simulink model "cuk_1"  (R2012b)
settings: Solver=ode45  StartTime=0.0  StopTime=10.0  RelTol=1e-3
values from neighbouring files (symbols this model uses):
  C1 = 200e-6    (= 0.0002)    [Cuk1.m]    (also in sepic1.m = 0.0001; sepic2.m = 0.0001; feder_masse_1.m = [1 0 0 0]; feder_masse_13.m = [1 0 0 0])
  C2 = C1    (= 0.0002)    [Cuk1.m]    (also in sepic1.m = 0.0001; sepic2.m = 0.0001; feder_masse_1.m = [0 0 1 0]; feder_masse_13.m = [0 0 1 0])
  f0 = 0.2e5    (= 20000)    [boost_up1.m]    (also in buck_boost1.m; buck_boost2.m; buck_down1.m; buck_down2.m)
  L1 = 0.0001    [Cuk1.m]    (also in sepic1.m = 5e-05; sepic2.m = 5e-05)
  L2 = L1    (= 0.0001)    [Cuk1.m]    (also in sepic1.m = 5e-05; sepic2.m = 5e-05)
  R = 5    [boost_up1.m]    (also in buck_boost1.m; buck_boost2.m; buck_down1.m = 2*Rmax,; buck_down2.m = 0.1*Rmax,)
  T = 1/f0    (= 5e-05)    [boost_up1.m]    (also in buck_boost1.m; buck_boost2.m; buck_down1.m; buck_down2.m)
  T1 = T-T2    (= 2.5e-05)    [buck_boost1.m]    (also in buck_boost2.m = 1e-05; sepic1.m = T-T2; sepic2.m = T-T2; unwucht_4.m = 500)
  Ui = 5    [boost_up1.m]    (also in buck_boost1.m; buck_boost2.m; buck_down1.m; buck_down2.m)

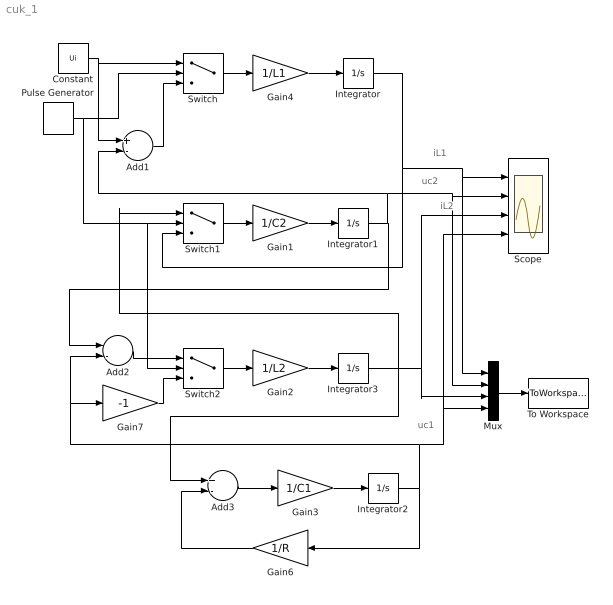
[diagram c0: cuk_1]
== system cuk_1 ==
  note: uc1
  note: iL2
  note: uc2
  note: iL1
  Add1 : Sum  Inputs=+-
  Add2 : Sum  Inputs=--
  Add3 : Sum  Inputs=+-
  Constant : Constant  Value=Ui
  Gain1 : Gain  Gain=1/C2
  Gain2 : Gain  Gain=1/L2
  Gain3 : Gain  Gain=1/C1
  Gain4 : Gain  Gain=1/L1
  Gain6 : Gain  Gain=1/R
  Gain7 : Gain  Gain=-1
  Integrator{,1..3} (4 alike) : Integrator
  Mux : Mux
  Pulse Generator : DiscretePulseGenerator  PulseType=Time based  Period=1/f0  PulseWidth=T1*100/T
  Scope : Scope  NumInputPorts=4
  Switch : Switch  Criteria=u2 > Threshold  Threshold=0.5  ZeroCross=off  SampleTime=0
  Switch1 : Switch  Criteria=u2 > Threshold  Threshold=0.5  ZeroCross=off  SampleTime=0
  Switch2 : Switch  Criteria=u2 > Threshold  Threshold=0.5  ZeroCross=off  SampleTime=0
  To Workspace : ToWorkspace  VariableName=y  SampleTime=-1  SaveFormat=Structure With Time
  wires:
  Constant/1 -> Add1/1, Switch/1
  Pulse Generator/1 -> Switch2/2, Switch1/2, Switch/2
  Add1/1 -> Switch/3
  Switch/1 -> Gain4/1
  Gain4/1 -> Integrator/1
  Switch1/1 -> Gain1/1
  Gain1/1 -> Integrator1/1
  Add2/1 -> Switch2/1
  Integrator1/1 -> Mux/2, Scope/2, Add1/2, Add2/1
  Switch2/1 -> Gain2/1
  Gain2/1 -> Integrator3/1
  Integrator3/1 -> Add3/1, Switch1/1, Mux/3, Scope/3
  Integrator/1 -> Mux/1, Scope/1, Switch1/3
  Add3/1 -> Gain3/1
  Gain3/1 -> Integrator2/1
  Gain6/1 -> Add3/2
  Gain7/1 -> Switch2/3
  Mux/1 -> To Workspace/1
  Integrator2/1 -> Mux/4, Scope/4, Gain7/1, Add2/2, Gain6/1
